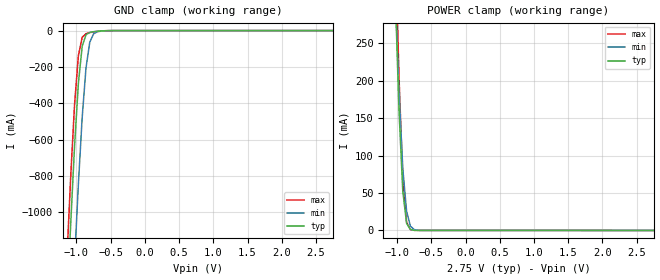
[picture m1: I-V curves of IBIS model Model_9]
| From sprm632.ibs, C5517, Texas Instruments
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| Model based on original model for IC33THYPD
|   Sub model IC33THY_PD_ON_COM_2P75
[model]   Model_9
|[Description]  [2.75V-INPUT-PD-X, COM]
|   PD,COM,
|[Input Load]   PD
|[Output Drive]
|Voltage   2.75V
|Mode   INPUT
Model_type   Input
Polarity   Non-Inverting
Vinl =  0.7
Vinh =  1.7
C_comp   0.88152539p  0.83844711p  0.88864286p
[Model Spec]
Vinl   0.7   0.7   0.7
Vinh   1.7   1.7   1.7
[Temperature Range]   25   105   -10
[Voltage Range]   2.75   2.475   3.025
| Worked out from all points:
|   GND clamp passes 1 mA (typ) near -0.59 V on its own axis
|   POWER clamp passes 1 mA (typ) near -0.79 V on its own axis
[POWER_clamp]
-2.75V    7.27A      6.262A     8.085A
-1.028V   318.4mA    321mA      393mA
-972.2mV  160.5mA    185.6mA    205.4mA
-916.7mV  52.38mA    82.72mA    68.25mA
-861.1mV  9.552mA    25.5mA     10.92mA
-805.6mV  1.329mA    5.828mA    1.207mA
-750mV    215.5uA    1.175mA    194.4uA
-638.9mV  63.87uA    77.5uA     93.3uA
2.75V     -84.09pA   -14.35uA   21.5uA
[GND_clamp]
-2.75V    -17A       -17.63A    -16.75A
-1.139V   -1.516A    -2.198A    -1.246A
-1.083V   -1.056A    -1.723A    -796.9mA
-1.028V   -635.2mA   -1.268A    -406.8mA
-972.2mV  -291mA     -845.8mA   -138.4mA
-916.7mV  -86.57mA   -479.1mA   -37.16mA
-861.1mV  -22.91mA   -206.5mA   -16.86mA
-805.6mV  -10.26mA   -63.94mA   -10.98mA
-750mV    -6.123mA   -17.61mA   -7.126mA
-694.4mV  -3.584mA   -6.2mA     -4.141mA
-638.9mV  -1.831mA   -2.781mA   -2.026mA
2.75V     61.47uA    35.47uA    92.23uA
